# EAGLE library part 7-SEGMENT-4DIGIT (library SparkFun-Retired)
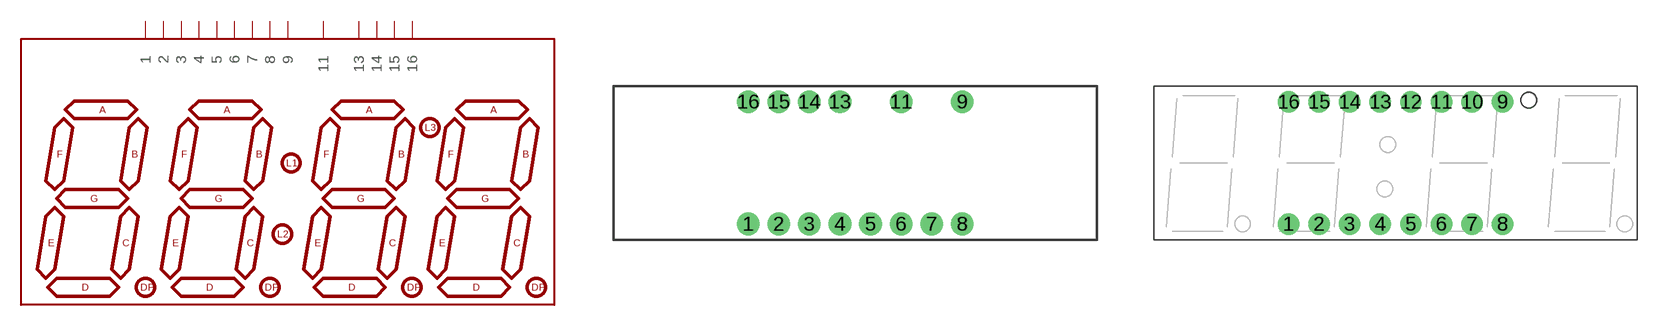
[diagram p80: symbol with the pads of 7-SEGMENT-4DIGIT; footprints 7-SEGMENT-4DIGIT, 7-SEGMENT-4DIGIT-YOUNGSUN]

Designator prefix -

## 7-SEGMENT-4DIGITPTH  [7-SEGMENT-4DIGIT]
1  1
2  2
3  3
4  4
5  5
6  6
7  7
8  8
9  9
11  11
13  13
14  14
15  15
16  16

## 7-SEGMENT-4DIGIT  [7-SEGMENT-4DIGIT-YOUNGSUN]
Pads as for 7-SEGMENT-4DIGIT

## 7-SEGMENT-4DIGITFOR_POGOBED_ONLY  [7-SEGMENT-4DIGIT_LONGPADS_FOR_POGOBED]
Pads as for 7-SEGMENT-4DIGIT

## Footprint 7-SEGMENT-4DIGIT (pad centres in mm)
drill 0.9 pad 1.88: 1 -8.89,-5.08; 2 -6.35,-5.08; 3 -3.81,-5.08; 4 -1.27,-5.08; 5 1.27,-5.08; 6 3.81,-5.08; 7 6.35,-5.08; 8 8.89,-5.08; 9 8.89,5.08; 11 3.81,5.08; 13 -1.27,5.08; 14 -3.81,5.08; 15 -6.35,5.08; 16 -8.89,5.08

## Footprint 7-SEGMENT-4DIGIT-YOUNGSUN (pad centres in mm)
This is a package for the 4-digit 7-segment RED LED from Young Sun.
drill 0.8 pad 1.778: 1 -8.89,-5.08; 2 -6.35,-5.08; 3 -3.81,-5.08; 4 -1.27,-5.08; 5 1.27,-5.08; 6 3.81,-5.08; 7 6.35,-5.08; 8 8.89,-5.08; 9 8.89,5.08; 10 6.35,5.08; 11 3.81,5.08; 12 1.27,5.08; 13 -1.27,5.08; 14 -3.81,5.08; 15 -6.35,5.08; 16 -8.89,5.08

## Footprint 7-SEGMENT-4DIGIT_LONGPADS_FOR_POGOBED (pad centres in mm)
drill 1.016 pad 1.88 long: 1 -8.89,-5.08; 2 -6.35,-5.08; 3 -3.81,-5.08; 4 -1.27,-5.08; 5 1.27,-5.08; 6 3.81,-5.08; 7 6.35,-5.08; 8 8.89,-5.08; 9 8.89,5.08; 11 3.81,5.08; 13 -1.27,5.08; 14 -3.81,5.08; 15 -6.35,5.08; 16 -8.89,5.08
